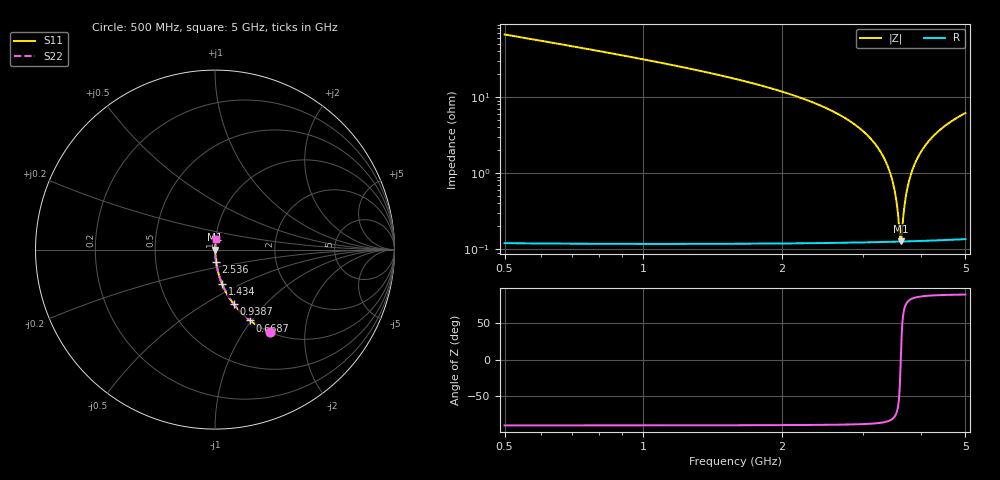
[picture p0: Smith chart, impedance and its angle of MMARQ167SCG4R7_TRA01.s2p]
! MMARQ167SCG4R7_TRA01  S-PARAMETER MODEL  ( General Type )
! Model Generated by TAIYO YUDEN Corporation (http://www.ty-top.com)
! Version 1.0
! TAIYO YUDEN Control No. 150305
! Copyright(c) 2015 TAIYO YUDEN CO.,LTD. All Rights Reserved.
! Product Description (link to TY-COMPAS)
! https://ds.yuden.co.jp/TYCOMPAS/or/detail?pn=MMARQ167SCG4R7BTRA01&u=M
! Products Name : Multilayer Ceramic Capacitors
! Characteristics :
!  Capacitance : 4.7 pF , Rated Voltage : 250V , TCC : CG / C0G
!  Case Size : 1.6 x 0.8 / 0.063 x 0.031 [mm/inch] , Thickness : 0.7 / 0.028 [mm/inch]
!  (Conditions: Temperature = 25 degC , DC Bias Current/Voltage = 0A / 0V)
! External Node Assignments :
!  1  o---| |---o  2
! GND o---------o GND
! Frequency Range : 500MHz  -  5GHz  [ 401 STEP ]
# MHz S RI R 50
! Freq[MHz].  S11 Real  S11 Imag  S21 Real  S21 Imag  S12 Real  S12 Imag  S22 Real  S22 Imag
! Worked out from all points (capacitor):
!   401 points, 500 MHz to 5 GHz, reference 50 ohm
!   read as one part in series: C = 4.68 pF near 522.5 MHz
!   lowest |Z| = 127 mohm at 3.616 GHz (marker M1)
!   series resonance near 3.62 GHz, so ESL is about 410 pH
!   S11 on the Smith chart (normalised r, x): 500 MHz: 1.00, -1.33; 668.8 MHz: 1.00, -0.98; 938.8 MHz: 1.00, -0.68; 1.434 GHz: 1.00, -0.40; 2.536 GHz: 1.00, -0.14; 5 GHz: 1.00, +0.12
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500  0.3082 -0.4609  0.6918 0.4609  0.6918 0.4609  0.3082 -0.4609
668.75  0.1949 -0.3949  0.8051 0.3949  0.8051 0.3949  0.1949 -0.3949
938.75  0.1033 -0.3026  0.8967 0.3026  0.8967 0.3026  0.1033 -0.3026
1253.75  0.0549 -0.2253  0.9451 0.2253  0.9451 0.2253  0.0549 -0.2253
1433.75  0.0395 -0.1918  0.9605 0.1918  0.9605 0.1918  0.0395 -0.1918
2007.5  0.0147 -0.1154  0.9853 0.1154  0.9853 0.1154  0.0147 -0.1154
2536.25  0.00582 -0.0678  0.9942 0.0678  0.9942 0.0678  0.00582 -0.0678
2750  0.00393 -0.052  0.9961 0.052  0.9961 0.052  0.00393 -0.052
3031.25  0.00234 -0.0334  0.9977 0.0334  0.9977 0.0334  0.00234 -0.0334
3245  0.00166 -0.0205  0.9983 0.0205  0.9983 0.0205  0.00166 -0.0205
3402.5  0.00138 -0.0116  0.9986 0.0116  0.9986 0.0116  0.00138 -0.0116
3503.75  0.00128 -0.00613  0.9987 0.00613  0.9987 0.00613  0.00128 -0.00613
3548.75  0.00126 -0.00374  0.9987 0.00374  0.9987 0.00374  0.00126 -0.00374
3593.75  0.00125 -0.00138  0.9987 0.00138  0.9987 0.00138  0.00125 -0.00138
3616.25  0.00125 -0.000206  0.9987 0.000206  0.9987 0.000206  0.00125 -0.000206
3638.75  0.00126 0.000956  0.9987 -0.000956  0.9987 -0.000956  0.00126 0.000956
3683.75  0.00127 0.00326  0.9987 -0.00326  0.9987 -0.00326  0.00127 0.00326
3728.75  0.00129 0.00553  0.9987 -0.00553  0.9987 -0.00553  0.00129 0.00553
3830  0.00138 0.0106  0.9986 -0.0106  0.9986 -0.0106  0.00138 0.0106
4010  0.00165 0.0192  0.9984 -0.0192  0.9984 -0.0192  0.00165 0.0192
4257.5  0.00223 0.0305  0.9978 -0.0305  0.9978 -0.0305  0.00223 0.0305
5000  0.00513 0.0613  0.9949 -0.0613  0.9949 -0.0613  0.00513 0.0613
